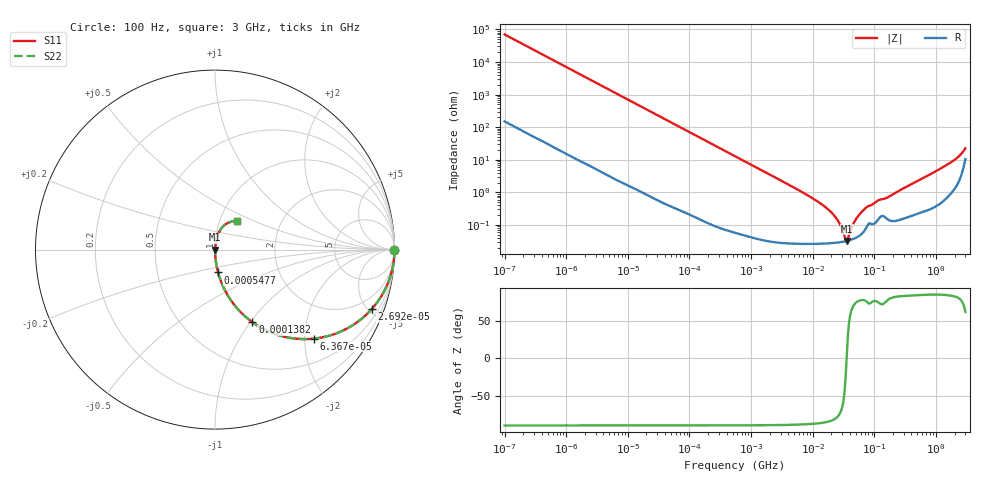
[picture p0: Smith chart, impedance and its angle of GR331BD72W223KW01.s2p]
!Murata Part Number: GR331BD72W223KW01
!These Parameters are Measured in Series Mode Connection
!Data Generated on Mar 13, 2026
!  o--ll--o
!Port1  Port2
!  o------o
!Operation Temp=25[degC], DC Bias Voltage=0[V]
!Freq. Start=100[Hz] Stop=3[GHz] 401[Steps]
# Hz S RI R 50
!Freq.(Hz) S11(Real) S11(Imag) S21(Real) S21(Imag) S12(Real) S12(Imag) S22(Real) S22(Imag)
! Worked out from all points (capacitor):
!   401 points, 100 Hz to 3 GHz, reference 50 ohm
!   read as one part in series: C = 22.7 nF near 109 Hz
!   lowest |Z| = 32.5 mohm at 35.63 MHz (marker M1)
!   series resonance near 35.46 MHz, so ESL is about 890 pH
!   S11 on the Smith chart (normalised r, x): 100 Hz: open; 26.92 kHz: 1.01, -5.25; 63.67 kHz: 1.01, -2.22; 138.2 kHz: 1.00, -1.02; 547.7 kHz: 1.00, -0.26; 3 GHz: 1.21, +0.40
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100  1 -0.00143  5.1e-06 0.00143  5.1e-06 0.00143  1 -0.00143
1788  0.9993 -0.0254  0.000702 0.0254  0.000702 0.0254  0.9993 -0.0254
8421  0.9857 -0.1177  0.0143 0.1177  0.0143 0.1177  0.9857 -0.1177
26919  0.8725 -0.3323  0.1275 0.3323  0.1275 0.3323  0.8725 -0.3323
31977  0.8293 -0.375  0.1707 0.375  0.1707 0.375  0.8293 -0.375
63668  0.5521 -0.4959  0.4479 0.4959  0.4479 0.4959  0.5521 -0.4959
138163  0.2087 -0.4049  0.7913 0.4049  0.7913 0.4049  0.2087 -0.4049
252400  0.0738 -0.2598  0.9262 0.2598  0.9262 0.2598  0.0738 -0.2598
547723  0.017 -0.1272  0.983 0.1272  0.983 0.1272  0.017 -0.1272
9794414  0.000308 -0.00671  0.9997 0.00671  0.9997 0.00671  0.000308 -0.00671
1.572531e7  0.000282 -0.00364  0.9997 0.00364  0.9997 0.00364  0.000282 -0.00364
2.21892e7  0.000285 -0.00195  0.9997 0.00195  0.9997 0.00195  0.000285 -0.00195
2.751729e7  0.000296 -0.00103  0.9997 0.00103  0.9997 0.00103  0.000296 -0.00103
3.268714e7  0.000313 -0.000328  0.9997 0.000328  0.9997 0.000328  0.000313 -0.000328
3.562563e7  0.000324 1.97e-05  0.9997 -1.97e-05  0.9997 -1.97e-05  0.000324 1.97e-05
3.882828e7  0.000338 0.000369  0.9997 -0.000369  0.9997 -0.000369  0.000338 0.000369
4.815176e7  0.000392 0.00127  0.9996 -0.00127  0.9996 -0.00127  0.000392 0.00127
6.794454e7  0.000647 0.00291  0.9994 -0.00291  0.9994 -0.00291  0.000647 0.00291
1.138854e8  0.00146 0.0054  0.9985 -0.0054  0.9985 -0.0054  0.00146 0.0054
1.751444e8  0.00144 0.00741  0.9986 -0.00741  0.9986 -0.00741  0.00144 0.00741
1.506733e9  0.0116 0.0687  0.9884 -0.0687  0.9884 -0.0687  0.0116 0.0687
3e9  0.1239 0.1574  0.8761 -0.1574  0.8761 -0.1574  0.1239 0.1574
